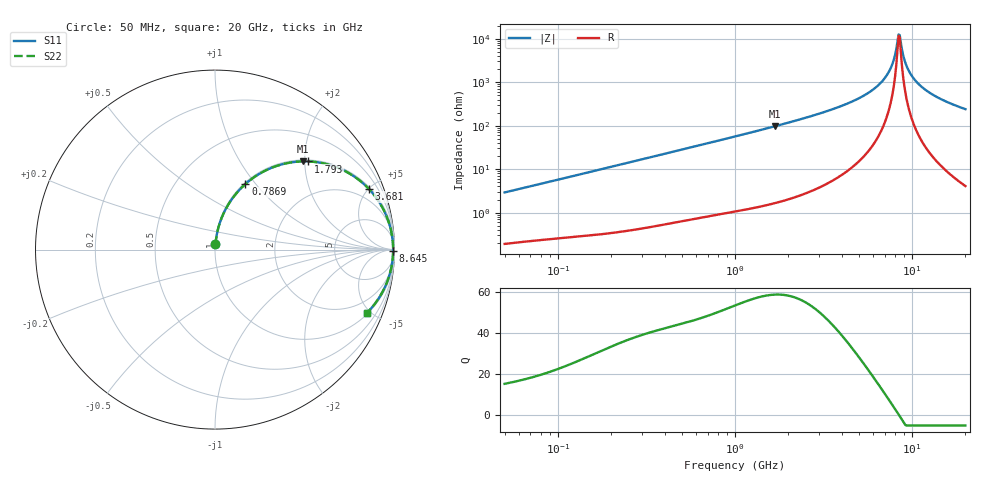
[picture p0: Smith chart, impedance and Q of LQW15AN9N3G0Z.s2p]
!Murata Part Number: LQW15AN9N3G0Z
!These Parameters are Measured in Series Mode Connection
!  o--[Z]--o
!Port1  Port2
!  o-------o
!Freq. Start=50[MHz] Stop=20[GHz], 401[Steps]
# Hz S RI R 50
!Freq.(Hz) S11(Real) S11(Imag) S21(Real) S21(Imag) S12(Real) S12(Imag) S22(Real) S22(Imag)
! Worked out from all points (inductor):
!   401 points, 50 MHz to 20 GHz, reference 50 ohm
!   read as one part in series: L = 9.2 nH near 51.52 MHz
!   highest Q = 58.7 at 1.689 GHz (marker M1), where L = 9.2 nH
!   self-resonance near 8.389 GHz
!   S11 on the Smith chart (normalised r, x): 50 MHz: 1.00, +0.06; 786.9 MHz: 1.02, +0.89; 1.793 GHz: 1.04, +2.08; 3.681 GHz: 1.12, +5.03; 8.645 GHz: open; 20 GHz: 1.08, -4.80
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5e7  0.00275 0.029  0.9973 -0.029  0.9973 -0.029  0.00275 0.029
1.364002e8  0.0088 0.0768  0.9912 -0.0768  0.9912 -0.0768  0.0088 0.0768
3.721004e8  0.0467 0.1992  0.9533 -0.1992  0.9533 -0.1992  0.0467 0.1992
7.868965e8  0.1691 0.365  0.8309 -0.365  0.8309 -0.365  0.1691 0.365
1e9  0.246 0.4214  0.754 -0.4214  0.754 -0.4214  0.246 0.4214
1.689197e9  0.4884 0.4914  0.5116 -0.4914  0.5116 -0.4914  0.4884 0.4914
1.793498e9  0.5204 0.4911  0.4796 -0.4911  0.4796 -0.4911  0.5204 0.4911
2.728004e9  0.7363 0.4313  0.2637 -0.4313  0.2637 -0.4313  0.7363 0.4313
3.680849e9  0.8579 0.3376  0.1421 -0.3376  0.1421 -0.3376  0.8579 0.3376
4.81993e9  0.9332 0.2337  0.0668 -0.2337  0.0668 -0.2337  0.9332 0.2337
5.856089e9  0.9677 0.1537  0.0323 -0.1537  0.0323 -0.1537  0.9677 0.1537
6.701223e9  0.9827 0.0973  0.0173 -0.0973  0.0173 -0.0973  0.9827 0.0973
7.442007e9  0.9896 0.0532  0.0104 -0.0532  0.0104 -0.0532  0.9896 0.0532
7.901521e9  0.9918 0.028  0.00825 -0.028  0.00825 -0.028  0.9918 0.028
8.264682e9  0.9925 0.00909  0.0075 -0.00909  0.0075 -0.00909  0.9925 0.00909
8.516016e9  0.9926 -0.00353  0.0074 0.00353  0.0074 0.00353  0.9926 -0.00353
8.644534e9  0.9925 -0.00984  0.00747 0.00984  0.00747 0.00984  0.9925 -0.00984
9.041845e9  0.9918 -0.0288  0.00817 0.0288  0.00817 0.0288  0.9918 -0.0288
9.457416e9  0.9904 -0.0477  0.0096 0.0477  0.0096 0.0477  0.9904 -0.0477
1.082228e10  0.9817 -0.1044  0.0183 0.1044  0.0183 0.1044  0.9817 -0.1044
1.396067e10  0.946 -0.2105  0.054 0.2105  0.054 0.2105  0.946 -0.2105
2e10  0.8482 -0.3505  0.1518 0.3505  0.1518 0.3505  0.8482 -0.3505
